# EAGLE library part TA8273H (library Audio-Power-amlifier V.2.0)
The TA8273H is 4 ch BTL audio power amplifier for car audio application. This IC can generate more high power: POUTMAX = 47 W as it is included the pure complementary PNP and NPN transistor output stage. It is designed low distortion ratio for 4 ch BTL audio power amplifier, built-in stand-by function, muting function, and diagnosis circuit which can detect output to VCC/GND short, output offset voltage and over voltage input mode. Additionally, the AUX amplifier and various kind of protector for car audio use are built-in.
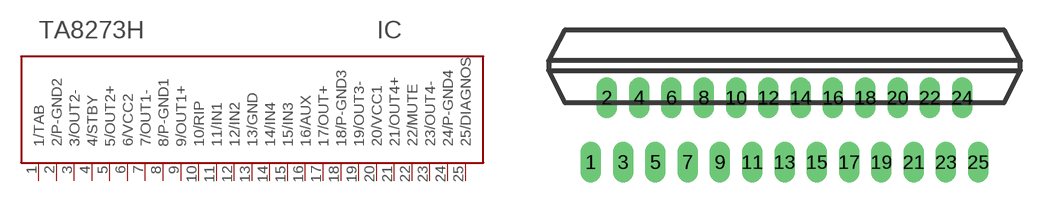
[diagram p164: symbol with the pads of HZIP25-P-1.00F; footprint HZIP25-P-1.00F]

Designator prefix IC

## TA8273H  [HZIP25-P-1.00F]
1  1/TAB
2  2/P-GND2  pwr
3  3/OUT2-  out
4  4/STBY  in
5  5/OUT2+  out
6  6/VCC2  pwr
7  7/OUT1-  out
8  8/P-GND1  pwr
9  9/OUT1+  out
10  10/RIP
11  11/IN1  in
12  12/IN2  in
13  13/GND  pwr
14  14/IN4  in
15  15/IN3  in
16  16/AUX  in
17  17/OUT+  out
18  18/P-GND3  pwr
19  19/OUT3-  out
20  20/VCC1  pwr
21  21/OUT4+  out
22  22/MUTE  in
23  23/OUT4-  out
24  24/P-GND4  pwr
25  25/DIAGNOS  out

## Footprint HZIP25-P-1.00F (pad centres in mm)
HZIP25-P-1.00F
drill 0.5 pad 1.27 long: 1 -12,-4; 2 -11,0; 3 -10,-4; 4 -9,0; 5 -8,-4; 6 -7,0; 7 -6,-4; 8 -5,0; 9 -4,-4; 10 -3,0; 11 -2,-4; 12 -1,0; 13 0,-4; 14 1,0; 15 2,-4; 16 3,0; 17 4,-4; 18 5,0; 19 6,-4; 20 7,0; 21 8,-4; 22 9,0; 23 10,-4; 24 11,0; 25 12,-4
